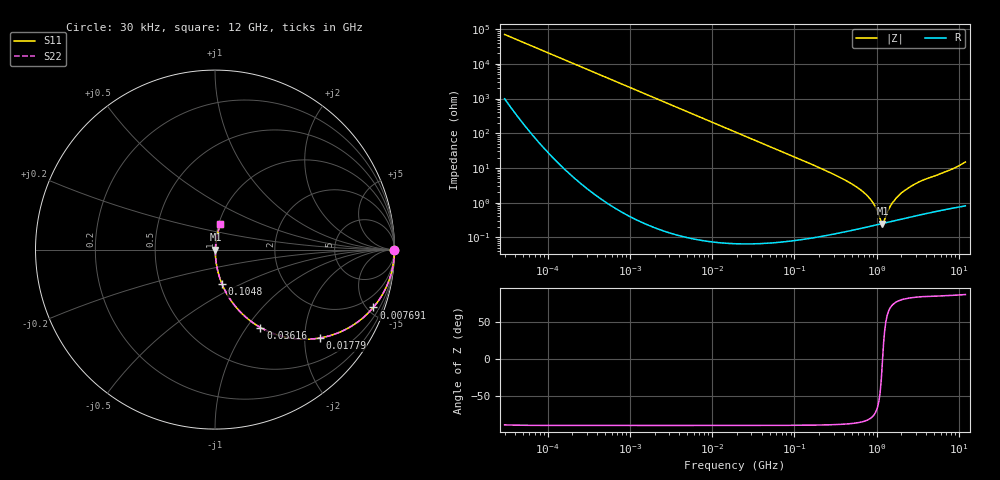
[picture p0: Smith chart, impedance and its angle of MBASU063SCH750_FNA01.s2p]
! MBASU063SCH750_FNA01  S-PARAMETER MODEL  ( General Type )
! Model Generated by TAIYO YUDEN Corporation (http://www.ty-top.com)
! Version 1.0
! TAIYO YUDEN Control No. 130801
! Copyright(c) 2013 TAIYO YUDEN CO.,LTD. All Rights Reserved.
! Product Description (link to TY-COMPAS)
! https://ds.yuden.co.jp/TYCOMPAS/or/detail?pn=MBASU063SCH750JFNA01&u=M
! Products Name : Multilayer Ceramic Capacitors
! Characteristics :
!  Capacitance : 75 pF , Rated Voltage : 50V , TCC : CH / C0H
!  Case Size : 0.6 x 0.3 / 0.024 x 0.012 [mm/inch] , Thickness : 0.3 / 0.012 [mm/inch]
!  (Conditions: Temperature = 25 degC , DC Bias Current/Voltage = 0A / 0V)
! External Node Assignments :
!  1  o---| |---o  2
! GND o---------o GND
! Frequency Range : 0.03MHz  -  12000MHz  [ 401 STEP ]
# MHz S RI R 50
! Freq[MHz].  S11 Real  S11 Imag  S21 Real  S21 Imag  S12 Real  S12 Imag  S22 Real  S22 Imag
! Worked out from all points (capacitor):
!   401 points, 30 kHz to 12 GHz, reference 50 ohm
!   read as one part in series: C = 75.6 pF near 32 kHz
!   lowest |Z| = 250 mohm at 1.177 GHz (marker M1)
!   series resonance near 1.18 GHz, so ESL is about 240 pH
!   S11 on the Smith chart (normalised r, x): 30 kHz: open; 7.691 MHz: 1.00, -5.48; 17.79 MHz: 1.00, -2.37; 36.16 MHz: 1.00, -1.16; 104.8 MHz: 1.00, -0.40; 12 GHz: 1.02, +0.30
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0.03  1 -0.00142  2.2e-05 0.00142  2.2e-05 0.00142  1 -0.00142
0.260295  0.9998 -0.0124  0.000158 0.0124  0.000158 0.0124  0.9998 -0.0124
2.258455  0.9886 -0.106  0.0114 0.106  0.0114 0.106  0.9886 -0.106
7.691429  0.8822 -0.3222  0.1178 0.3222  0.1178 0.3222  0.8822 -0.3222
11.69699  0.7641 -0.4244  0.2359 0.4244  0.2359 0.4244  0.7641 -0.4244
17.78857  0.5835 -0.4927  0.4165 0.4927  0.4165 0.4927  0.5835 -0.4927
18.97367  0.5518 -0.497  0.4482 0.497  0.4482 0.497  0.5518 -0.497
36.16215  0.2532 -0.4343  0.7468 0.4343  0.7468 0.4343  0.2532 -0.4343
58.65857  0.1142 -0.317  0.8858 0.317  0.8858 0.317  0.1142 -0.317
104.8152  0.039 -0.1914  0.961 0.1914  0.961 0.1914  0.039 -0.1914
164.6252  0.0164 -0.1233  0.9836 0.1233  0.9836 0.1233  0.0164 -0.1233
393.2198  0.00366 -0.0474  0.9963 0.0474  0.9963 0.0474  0.00366 -0.0474
658.7456  0.00231 -0.0219  0.9977 0.0219  0.9977 0.0219  0.00231 -0.0219
880.5704  0.00225 -0.0106  0.9978 0.0106  0.9978 0.0106  0.00225 -0.0106
970.0175  0.0023 -0.00704  0.9977 0.00704  0.9977 0.00704  0.0023 -0.00704
1103.571  0.00242 -0.00242  0.9976 0.00242  0.9976 0.00242  0.00242 -0.00242
1177.092  0.0025 -7.87e-05  0.9975 7.87e-05  0.9975 7.87e-05  0.0025 -7.87e-05
1255.512  0.00259 0.0021  0.9974 -0.0021  0.9974 -0.0021  0.00259 0.0021
1428.372  0.00282 0.00648  0.9972 -0.00648  0.9972 -0.00648  0.00282 0.00648
1848.769  0.00343 0.0155  0.9966 -0.0155  0.9966 -0.0155  0.00343 0.0155
2635.962  0.00474 0.0294  0.9953 -0.0294  0.9953 -0.0294  0.00474 0.0294
12000  0.0291 0.1431  0.9709 -0.1431  0.9709 -0.1431  0.0291 0.1431
